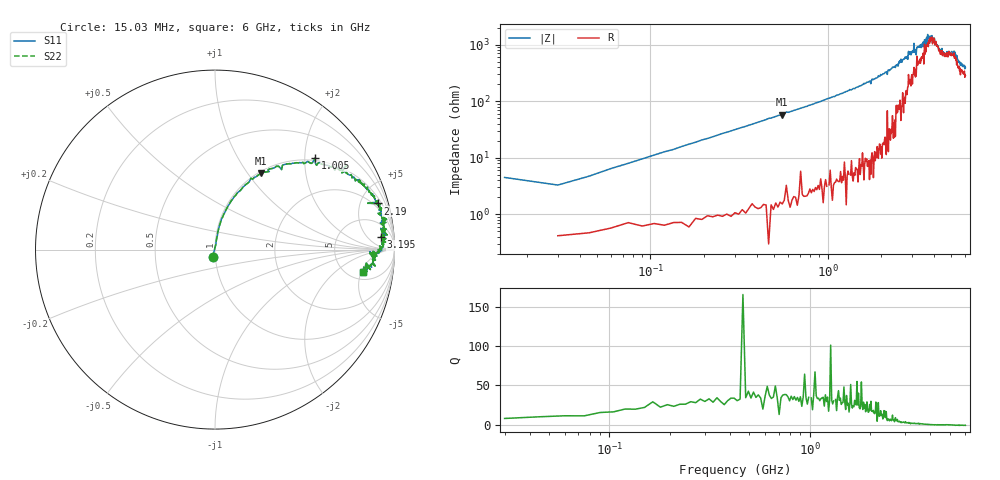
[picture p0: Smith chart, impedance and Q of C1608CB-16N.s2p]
!	Network	Analyzer	HP8753E.07.74:	Oct	30	2002	Serial	No.	JP38451487
!	Hewlett-Packard
!	28	Aug	2009	7:55:30
!	Frequency	S11	S21	S12	S22
#	HZ	S	RI	R	50
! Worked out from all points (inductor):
!   400 points, 15.03 MHz to 6 GHz, reference 50 ohm
!   read as one part in series: L = 16.9 nH near 45.03 MHz
!   highest Q = 36.2 at 555 MHz (marker M1), where L = 16.6 nH
!   self-resonance near 3.989 GHz
!   S11 on the Smith chart (normalised r, x): 15.03 MHz: 0.97, -0.09; 1.005 GHz: 0.94, +2.24; 2.19 GHz: 1.51, +6.86; 3.195 GHz: 14, +13; 6 GHz: 6.68, -5.46
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1.502992e7  -0.0139 -0.0439  1.01 0.0439  1.01 0.0439  -0.0139 -0.0439
3.002985e7  0.00544 0.0324  0.995 -0.0324  0.995 -0.0324  0.00544 0.0324
9.002955e7  0.0152 0.0938  0.985 -0.0938  0.985 -0.0938  0.0152 0.0938
1.95029e8  0.048 0.195  0.952 -0.195  0.952 -0.195  0.048 0.195
5.550272e8  0.257 0.424  0.743 -0.424  0.743 -0.424  0.257 0.424
1.005025e9  0.558 0.51  0.442 -0.51  0.442 -0.51  0.558 0.51
1.020025e9  0.559 0.482  0.441 -0.482  0.441 -0.482  0.559 0.482
2.01002e9  0.881 0.298  0.119 -0.298  0.119 -0.298  0.881 0.298
2.190019e9  0.906 0.257  0.0944 -0.257  0.0944 -0.257  0.906 0.257
3.015015e9  0.954 0.114  0.0455 -0.114  0.0455 -0.114  0.954 0.114
3.075015e9  0.959 0.0811  0.0411 -0.0811  0.0411 -0.0811  0.959 0.0811
3.165014e9  0.924 0.119  0.0758 -0.119  0.0758 -0.119  0.924 0.119
3.195014e9  0.924 0.0686  0.0759 -0.0686  0.0759 -0.0686  0.924 0.0686
3.495013e9  0.943 0.0838  0.0571 -0.0838  0.0571 -0.0838  0.943 0.0838
3.675012e9  0.953 0.0423  0.0465 -0.0423  0.0465 -0.0423  0.953 0.0423
3.705011e9  0.927 0.0426  0.0726 -0.0426  0.0726 -0.0426  0.927 0.0426
4.00501e9  0.929 -0.00644  0.0707 0.00644  0.0707 0.00644  0.929 -0.00644
4.03501e9  0.909 0.000274  0.0913 -0.000274  0.0913 -0.000274  0.909 0.000274
4.425008e9  0.902 -0.0362  0.0985 0.0362  0.0985 0.0362  0.902 -0.0362
4.455008e9  0.87 -0.0249  0.13 0.0249  0.13 0.0249  0.87 -0.0249
5.010005e9  0.886 -0.0343  0.114 0.0343  0.114 0.0343  0.886 -0.0343
6e9  0.827 -0.123  0.173 0.123  0.173 0.123  0.827 -0.123
